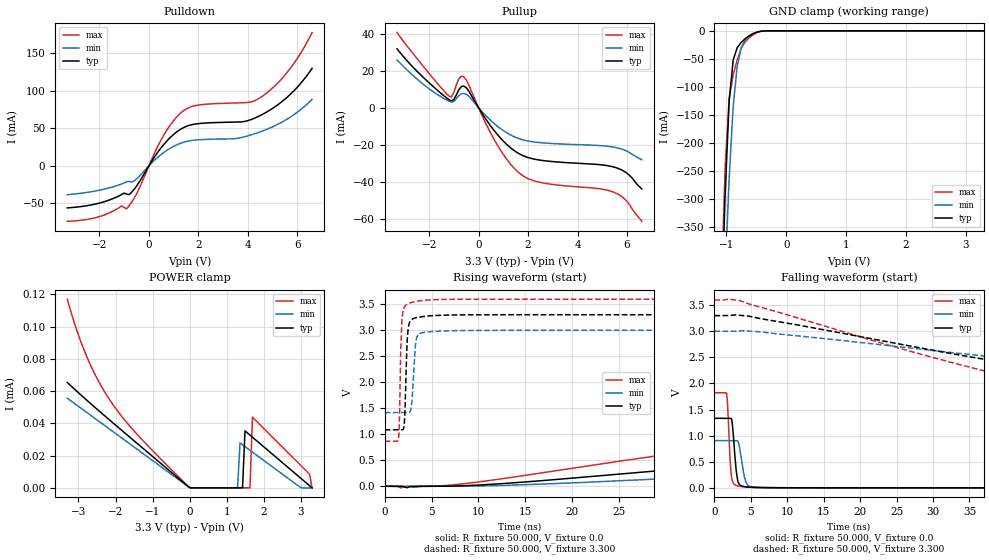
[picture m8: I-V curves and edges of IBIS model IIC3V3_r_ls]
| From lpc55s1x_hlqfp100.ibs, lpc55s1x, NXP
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|   Model IIC3V3_r_ls
[Model] IIC3V3_r_ls
Model_type I/O
Polarity   Non-Inverting
Enable   Active-Low
Vinl =  0.990V
Vinh =  2.310V
Vmeas =  1.650V
Cref =  0.0F
Rref =  100.000
Vref =  0.0V
C_comp   2.367pF   2.322pF   2.392pF
C_comp_pullup   0.514pF   0.422pF   0.587pF
C_comp_pulldown   1.565pF   1.480pF   1.637pF
[Model Spec]
Vinh   2.310V   2.100V   2.520V
Vinl   0.990V   0.900V   1.080V
Vmeas   1.650V   1.500V   1.800V
Vref   0.0V   0.0V   0.0V
Cref   0.0F   0.0F   0.0F
Rref   100.000   100.000   100.000
[Temperature Range]   25.000   0.125k   -40.000
[Voltage Range]   3.300V   3.000V   3.600V
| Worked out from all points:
|   slope of the pulldown table from 0 to 0.495 V, typ, clamps not added: 20.4 ohm
|   slope of the pullup table from 0 to 0.495 V, typ, clamps not added: 49.8 ohm
|   GND clamp passes 1 mA (typ) near -0.43 V on its own axis
|   rising waveform, R_fixture 50.000, V_fixture 0.0: 20-80 % time 64.7ns typ, 78.1ns min, 51.2ns max; typ from 0 V to 1.32 V
|   rising waveform, R_fixture 50.000, V_fixture 3.300: 20-80 % time 237ps typ, 323ps min, 203ps max; typ from 1.08 V to 3.3 V
|   falling waveform, R_fixture 50.000, V_fixture 0.0: 20-80 % time 477ps typ, 654ps min, 378ps max; typ from 1.33 V to 0 V
|   falling waveform, R_fixture 50.000, V_fixture 3.300: 20-80 % time 50.7ns typ, 68.5ns min, 38.4ns max; typ from 3.3 V to 1.09 V
[Pulldown]
|Voltage   I(typ)   I(min)   I(max)
-3.3V     -56mA      -38.4mA    -73.87mA
-2.1V     -50.37mA   -33.07mA   -68.52mA
-1.1V     -38.15mA   -24.11mA   -53.37mA
-900mV    -37.61mA   -21.16mA   -57.18mA
-500mV    -26.92mA   -17.4mA    -37.43mA
500mV     24.51mA    15.34mA    35.14mA
1.2V      47.07mA    29.16mA    67.89mA
1.9V      55.94mA    34.55mA    80.54mA
3.8V      58.93mA    38.31mA    84.23mA
4.5V      67.15mA    45.39mA    91.04mA
5.6V      91.85mA    62.59mA    125mA
6.6V      130mA      88.72mA    177.8mA
[Pullup]
|Voltage   I(typ)   I(min)   I(max)
-3.3V     31.77mA    25.72mA    40.57mA
-2.2V     15.94mA    12.27mA    21.75mA
-1.2V     4.452mA    3.6mA      6.337mA
-1.1V     3.726mA    3.058mA    5.816mA
-800mV    9.696mA    6.594mA    15.7mA
-600mV    11.73mA    7.748mA    16.71mA
700mV     -13.46mA   -9.282mA   -18.76mA
1.7V      -25.21mA   -16.93mA   -35.78mA
2.6V      -28.44mA   -18.91mA   -40.52mA
5.5V      -32.06mA   -21.31mA   -45.71mA
6V        -35.26mA   -23.41mA   -50.46mA
6.6V      -43.76mA   -28.06mA   -61.21mA
[GND_clamp]
|Voltage   I(typ)   I(min)   I(max)
-3.3V     -10.05A    -9.18A     -11.33A
-1.089V   -516.5mA   -633.7mA   -475mA
-1.022V   -291.9mA   -436.3mA   -243.2mA
-955mV    -126mA     -264mA     -120.7mA
-888mV    -52.17mA   -135.6mA   -79.12mA
-821mV    -30.44mA   -63.69mA   -52.12mA
-754mV    -20.67mA   -30.69mA   -31.05mA
-687mV    -14.19mA   -15.97mA   -19.65mA
-553mV    -5.021mA   -4.512mA   -7.044mA
-419mV    -659.6uA   -714.3uA   -896.4uA
-285mV    -20.38uA   -37.42uA   -22.84uA
3.3V      0A         0A         0A
[POWER_clamp]
|Voltage   I(typ)   I(min)   I(max)
-3.3V     65.36uA    55.62uA    117.1uA
-2.797V   54.84uA    47.15uA    82.63uA
-2.194V   42.78uA    37.02uA    55.95uA
-50mV     976.9nA    858.9nA    1.15uA
1.29V     0A         0A         0A
1.357V    0A         27.85uA    0A
1.424V    0A         26.71uA    0A
1.491V    35.37uA    25.58uA    0A
1.625V    32.75uA    23.31uA    0A
1.692V    31.44uA    22.17uA    43.84uA
3.233V    1.309uA    0A         8.433uA
3.3V      0A         0A         0A
[Ramp]
| variable   typ   min   max
dV/dt_r   0.795/64.660n   0.534/78.103n   1.092/51.208n
dV/dt_f   1.328/50.715n   0.947/68.465n   1.640/38.387n
R_load = 50.000
[Rising Waveform]
R_fixture= 50.000
V_fixture= 0.0
V_fixture_min= 0.0
V_fixture_max= 0.0
|time   V(typ)   V(min)   V(max)
0s        10.23nV    71.93nV    30.73nV
1.74ns    77.62uV    89.62nV    -30.99mV
8.05ns    6.834mV    602.5uV    40.19mV
41.01ns   473.8mV    241.1mV    856.9mV
71.47ns   827.6mV    470.3mV    1.449V
84.41ns   980mV      550.4mV    1.616V
101.9ns   1.142V     652.5mV    1.725V
123.9ns   1.243V     768.4mV    1.782V
155.2ns   1.3V       849.3mV    1.81V
200ns     1.325V     889.4mV    1.821V
[Rising Waveform]
R_fixture= 50.000
V_fixture= 3.300
V_fixture_min= 3.000
V_fixture_max= 3.600
|time   V(typ)   V(min)   V(max)
0s        1.085V     1.417V     866.6mV
1.47ns    1.085V     1.417V     919.2mV
1.55ns    1.085V     1.417V     1.177V
1.77ns    1.085V     1.417V     2.998V
1.99ns    1.102V     1.417V     3.399V
2.57ns    3.107V     1.417V     3.519V
2.87ns    3.206V     1.569V     3.536V
3.36ns    3.243V     2.815V     3.557V
4.43ns    3.271V     2.966V     3.58V
200ns     3.3V       3V         3.6V
[Falling Waveform]
R_fixture= 50.000
V_fixture= 0.0
V_fixture_min= 0.0
V_fixture_max= 0.0
|time   V(typ)   V(min)   V(max)
0s        1.333V     906.1mV    1.824V
1.66ns    1.333V     906.1mV    1.805V
1.83ns    1.333V     906.1mV    1.514V
2.18ns    1.334V     906.1mV    454.3mV
2.46ns    1.206V     906.1mV    128.9mV
2.87ns    485.8mV    906.1mV    52.76mV
3.18ns    146.1mV    897.6mV    37.4mV
4.09ns    24.67mV    221.7mV    17.98mV
4.48ns    17.61mV    66.68mV    13.7mV
200ns     187.6nV    456.6nV    118.2nV
[Falling Waveform]
R_fixture= 50.000
V_fixture= 3.300
V_fixture_min= 3.000
V_fixture_max= 3.600
|time   V(typ)   V(min)   V(max)
0s        3.3V       3V         3.6V
3.33ns    3.308V     3.007V     3.594V
29.21ns   2.656V     2.643V     2.527V
48.9ns    2.199V     2.361V     1.847V
57.25ns   2.031V     2.256V     1.262V
66.1ns    1.793V     2.154V     1.024V
77.89ns   1.378V     2.028V     930.2mV
95.24ns   1.184V     1.734V     887.8mV
126.6ns   1.106V     1.493V     870.4mV
200ns     1.086V     1.422V     866.8mV
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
